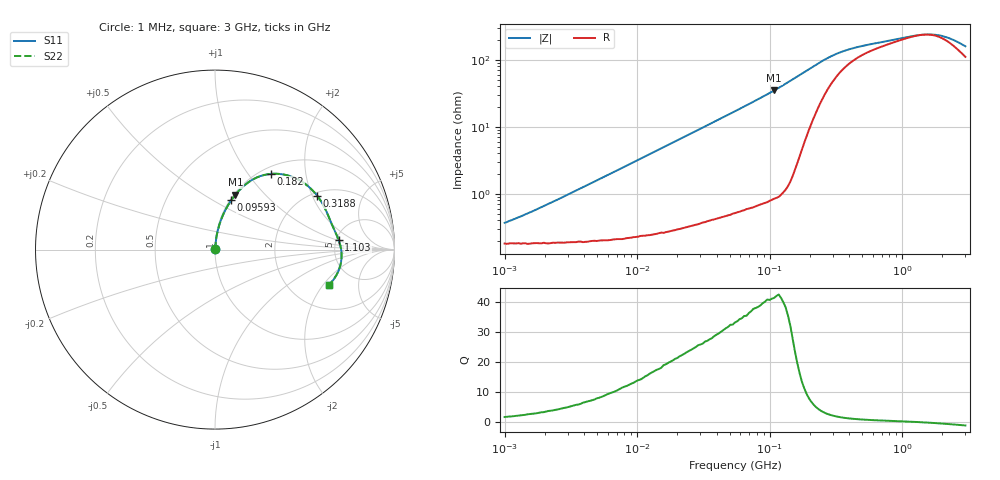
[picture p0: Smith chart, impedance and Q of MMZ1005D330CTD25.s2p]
! S-Parameter Data Generated by TDK Corporation
! Copyright(C) 2025 TDK Corporation.
! All Rights Reserved.
! TDK P/N: MMZ1005D330CTD25 (Chip Bead)
! Property: |Z|=33ohm at 100MHz
! Size(LxWxT): 1x0.5x0.5mm
! Model Type: s2p (Touchstone File Format Version 1.0)
! Frequency: DC=Yes Start=1MHz Stop=3000MHz 202points Log-sweep
! Model Generated on Feb. 6, 2025
! Terms and conditions regarding TDK Simulation Models:
! 1)This simulation model is being provided solely for informational
!  purposes. Please refer to the specifications of the products in
!  terms of detailed characteristics of such products.
! 2)In no event shall TDK Corporation of any of its subsidiaries be
!  liable for any loss or damage arising, directly or indirectly,
!  from any information contained in this simulation model, including,
!  but not limited to loss or damages arising from any inaccuracies,
!  omissions or errors in connection with such information.
! 3)Any and all copyrights on this simulation model are owned by
!  TDK Corporation.  Duplication or redistribution of this simulation
!  model without prior written permission from TDK Corporation
!  is prohibited.
! 4)This simulation model is subject to any modification or change
!  without any prior notice.
! 5)Neither TDK Corporation nor any of its subsidiaries shall make any
!  warranty, express or implied, including but not limited to the
!  correctness, implied warranties of merchantability and fitness for
!  a particular purpose with respect to this simulation models.
! 6)The use of this simulation model shall be deemed to have consented
!  to the terms and conditions hereof.
! Port Assignments:
!  1 ---@@@--- 2
! Applicable Conditions:
!  Temperature = 25 degC
!  DC Bias Current = 0 A
!  Small Signal Operation
# Hz S MA R 50
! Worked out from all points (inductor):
!   201 points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, 1 MHz to 3 GHz, reference 50 ohm
!   read as one part in series: L = 50.6 nH near 1.751 MHz
!   highest Q = 41.3 at 108.2 MHz (marker M1), where L = 51.2 nH
!   self-resonance near 1.443 GHz
!   S11 on the Smith chart (normalised r, x): 1 MHz: 1.00, +0.01; 95.93 MHz: 1.01, +0.61; 182 MHz: 1.11, +1.30; 318.8 MHz: 2.12, +2.18; 1.103 GHz: 5.25, +1.07; 3 GHz: 3.21, -2.28
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1000000  0.003667 60.4  0.9982 -0.2  0.9982 -0.2  0.003667 60.4
1616692  0.005425 70.1  0.9982 -0.3  0.9982 -0.3  0.005425 70.1
3900413  0.01244 80.6  0.998 -0.7  0.998 -0.7  0.01244 80.6
1.461624e7  0.0456 84.2  0.9964 -2.6  0.9964 -2.6  0.0456 84.2
3.00453e7  0.09265 82.5  0.9921 -5.3  0.9921 -5.3  0.09265 82.5
5.477226e7  0.1669 78.7  0.9809 -9.6  0.9809 -9.6  0.1669 78.7
7.544761e7  0.2286 75.3  0.9675 -13.2  0.9675 -13.2  0.2286 75.3
9.593103e7  0.2895 71.8  0.9501 -16.8  0.9501 -16.8  0.2895 71.8
1.081723e8  0.3261 69.6  0.9375 -19.0  0.9375 -19.0  0.3261 69.6
1.431579e8  0.4306 62.7  0.8893 -25.5  0.8893 -25.5  0.4306 62.7
1.820241e8  0.5254 53.4  0.8062 -31.6  0.8062 -31.6  0.5254 53.4
2.136344e8  0.5777 45.8  0.7264 -34.7  0.7264 -34.7  0.5777 45.8
2.609752e8  0.6219 36.0  0.6171 -36.3  0.6171 -36.3  0.6219 36.0
3.188066e8  0.6435 27.9  0.526 -34.9  0.526 -34.9  0.6435 27.9
3.741707e8  0.6516 22.9  0.4731 -32.4  0.4731 -32.4  0.6516 22.9
4.570858e8  0.6572 18.0  0.4266 -28.5  0.4266 -28.5  0.6572 18.0
8.005644e8  0.6749 9.0  0.3496 -17.5  0.3496 -17.5  0.6749 9.0
1.10276e9  0.6911 4.4  0.3155 -9.7  0.3155 -9.7  0.6911 4.4
1.519029e9  0.7045 -1.0  0.2959 2.3  0.2959 2.3  0.7045 -1.0
1.855641e9  0.706 -5.0  0.303 11.8  0.303 11.8  0.706 -5.0
2.266846e9  0.6984 -9.7  0.3333 20.8  0.3333 20.8  0.6984 -9.7
3e9  0.6634 -17.5  0.4179 28.5  0.4179 28.5  0.6634 -17.5
